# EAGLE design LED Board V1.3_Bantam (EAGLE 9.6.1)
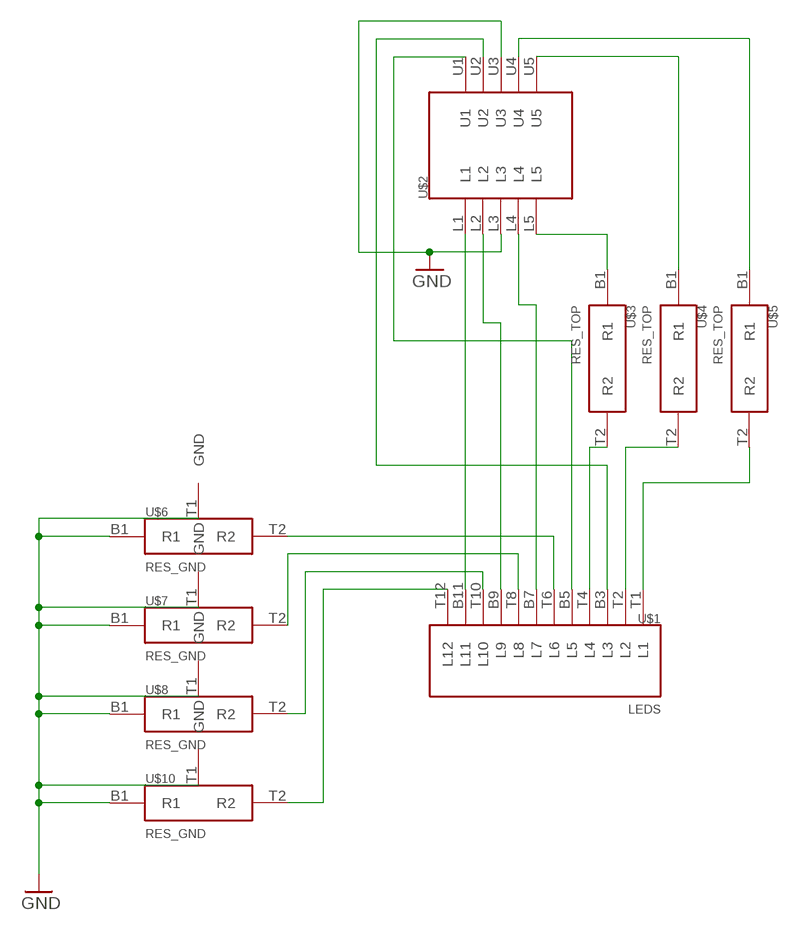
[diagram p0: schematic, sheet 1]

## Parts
U$1  LEDS  [F_LEDS]
U$2  2X5  [F_2X5]
U$3  RES_TOP  [F_RES]
U$4  RES_TOP  [F_RES]
U$5  RES_TOP  [F_RES]
U$6  RES_GND  [F_RES_GND]
U$7  RES_GND  [F_RES_GND]
U$8  RES_GND  [F_RES_GND]
U$10  RES_GND  [F_RES_GND]

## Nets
GND: U$2.L3 U$2.U3 U$6.B1(R1) U$6.T1(GND) U$7.B1(R1) U$7.T1(GND) U$8.B1(R1) U$8.T1(GND) U$10.B1(R1) U$10.T1(GND)
N$1: U$1.T12(L12) U$10.T2(R2)
N$2: U$1.T10(L10) U$8.T2(R2)
N$3: U$1.T8(L8) U$7.T2(R2)
N$4: U$1.T6(L6) U$6.T2(R2)
N$5: U$1.T4(L4) U$3.T2(R2)
N$6: U$1.T2(L2) U$4.T2(R2)
N$7: U$1.T1(L1) U$5.T2(R2)
N$8: U$1.B11(L11) U$2.L1
N$9: U$1.B9(L9) U$2.L2
N$10: U$1.B7(L7) U$2.L4
N$11: U$2.L5 U$3.B1(R1)
N$12: U$2.U5 U$4.B1(R1)
N$13: U$2.U4 U$5.B1(R1)
N$14: U$1.B5(L5) U$2.U1
N$15: U$1.B3(L3) U$2.U2

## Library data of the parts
U$1 = OpenMMS_Bantam:LEDS
U$2 = OpenMMS_Bantam:2X5
U$3-U$5 = OpenMMS_Bantam:RES_TOP
U$6-U$8 U$10 = OpenMMS_Bantam:RES_GND

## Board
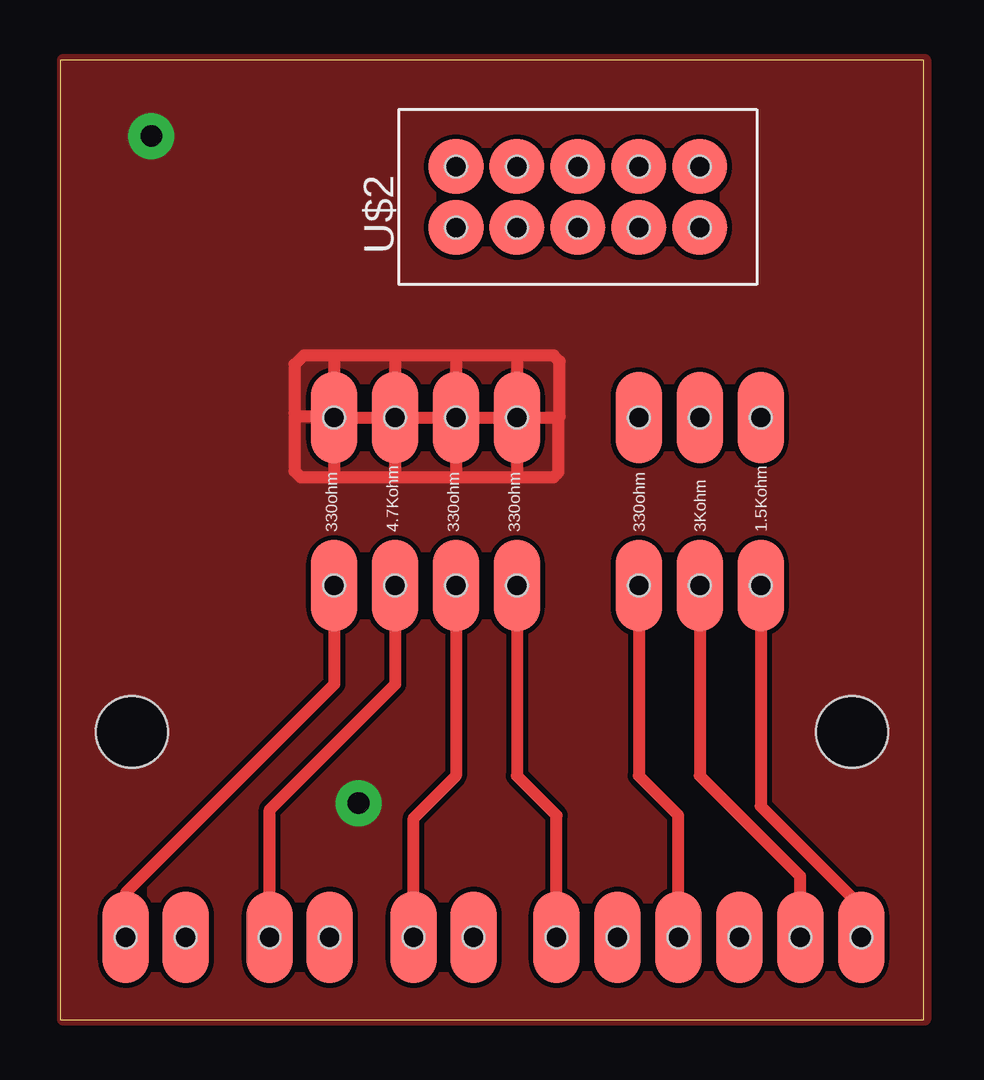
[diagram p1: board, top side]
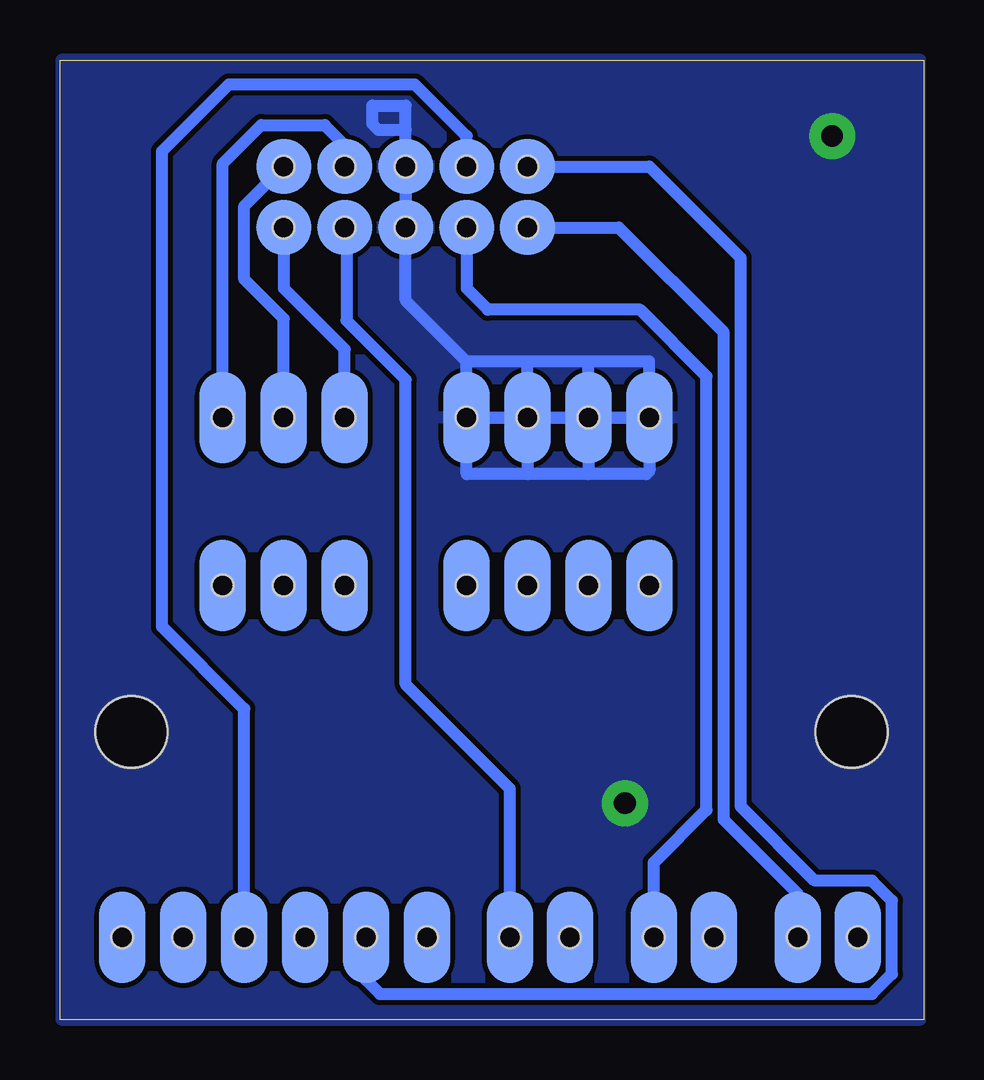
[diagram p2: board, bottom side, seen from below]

Size 36 x 40 mm. Coordinates in mm from the lower left corner, seen from the top.
Outline: 0,0 36,0 36,40 0,40 0,0
Copper layers (1*16): Top 0.035mm / dielectric 1.5mm / Bottom 0.035mm
Design rules "OpenMMS_Bantam": minimum track width 20mil, minimum drill 0.9mm, track to track 8mil, track to pad 8mil, pad to pad 8mil, via to via 8mil, smd to smd 8mil, copper to edge 0mil, drill to drill 0mil, minimum pad ring 20mil, minimum via ring 20mil, stop-mask expansion 4mil, vias tented up to drill 0mil, thermal gap 8mil
Holes 3 mm at 33.02,11.99 3,11.99

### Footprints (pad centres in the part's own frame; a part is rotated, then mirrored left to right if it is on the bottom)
F_LEDS = smd 1.93 x 3.81 bottom: B1 10.16,0; B2 7.62,0; B3 5.08,0; B4 2.54,0; B5 0,0; B6 -2.54,0; B7 -6,0; B8 -8.5,0; B9 -12,0; B10 -14.5,0; B11 -18,0; B12 -20.5,0 | smd 1.93 x 3.81: T1 10.16,0; T2 7.62,0; T3 5.08,0; T4 2.54,0; T5 0,0; T6 -2.54,0; T7 -6,0; T8 -8.5,0; T9 -12,0; T10 -14.5,0; T11 -18,0; T12 -20.5,0 | hole 0.9: 10.16,0; 7.62,0; 5.08,0; 2.54,0; 0,0; -2.54,0; -6,0; -8.5,0; -12,0; -14.5,0; -18,0; -20.5,0
F_2X5 = smd 2.286 x 2.286: B1 -5.08,-1.27; B2 -2.54,-1.27; B3 0,-1.27; B4 2.54,-1.27; B5 5.08,-1.27; B6 5.08,1.27; B7 2.54,1.27; B8 0,1.27; B9 -2.54,1.27; B20 -5.08,1.27 | smd 2.286 x 2.286 bottom: L1 -5.08,-1.27; L2 -2.54,-1.27; L3 0,-1.27; L4 2.54,-1.27; L5 5.08,-1.27; U1 -5.08,1.27; U2 -2.54,1.27; U3 0,1.27; U4 2.54,1.27; U5 5.08,1.27 | hole 0.9: -5.08,-1.27; -2.54,-1.27; 0,-1.27; 2.54,-1.27; 5.08,-1.27; 5.08,1.27; 2.54,1.27; 0,1.27; -2.54,1.27; -5.08,1.27
F_RES = smd 1.93 x 3.81 bottom: B1 0,3.5; B2 0,-3.5 | smd 1.93 x 3.81: T1 0,3.5; T2 0,-3.5 | hole 0.9: 0,3.5; 0,-3.5
F_RES_GND = smd 1.93 x 3.81 bottom: B1 0,3.5; B2 0,-3.5 | smd 1.93 x 3.81: T1 0,3.5; T2 0,-3.5 | hole 0.9: 0,3.5; 0,-3.5

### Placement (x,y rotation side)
U$1  23.24,3.43 0 top
U$2  21.59,34.29 0 top
U$3  24.13,21.59 0 top
U$4  26.67,21.59 0 top
U$5  29.21,21.59 0 top
U$6  19.05,21.59 0 top
U$7  16.51,21.59 0 top
U$8  13.97,21.59 0 top
U$10  11.43,21.59 0 top

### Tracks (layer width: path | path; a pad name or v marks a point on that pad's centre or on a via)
GND  (via drill 0.9)
  Top 0.508: 13.27,25.09 U$10.T1 11.43,22.61 | 13.27,25.09 U$8.T1 | U$8.T1 15.81,25.09 | 15.81,25.09 U$7.T1 | U$7.T1 18.35,25.09 | 18.35,25.09 U$6.T1 | U$6.T1 20.77,25.09 | 20.77,25.09 20.83,25.15 20.83,27.43 20.57,27.69 19.05,27.69 | 19.05,27.69 16.51,27.69 | 16.51,27.69 13.97,27.69 | 13.97,27.69 11.43,27.69 | 11.43,27.69 10.16,27.69 9.78,27.3 9.78,25.27 | 9.78,25.27 9.91,25.15 10.67,25.15 10.73,25.09 10.73,25.38 11.43,26.09 11.43,27.69 | 9.78,25.27 9.78,22.86 10.03,22.61 11.43,22.61 | 11.43,22.61 13.97,22.61 | 13.97,22.61 16.51,22.61 | 16.51,22.61 19.05,22.61 | 19.05,22.61 20.57,22.61 20.77,22.8 20.77,25.09 | 13.27,25.09 13.27,25.38 13.97,26.09 13.97,27.69 | U$8.T1 13.97,22.61 | 15.81,25.09 15.81,25.38 16.51,26.09 16.51,27.69 | U$7.T1 16.51,22.61 | 18.35,25.09 18.35,25.38 19.05,26.09 19.05,27.69 | U$6.T1 19.05,22.61
  Bottom 0.508: 19.05,27.43 U$6.T1 U$7.T1 | 19.05,27.43 21.59,29.97 21.59,32.02 20.89,32.73 20.89,33.02 | U$10.T1 11.43,27.43 13.97,27.43 | 13.97,27.43 16.51,27.43 | 16.51,27.43 19.05,27.43 | U$8.T1 13.97,27.43 | U$7.T1 16.51,27.43 | U$2.L3 U$2.U3 21.59,37.08 | U$10.T1 11.43,22.86 11.56,22.73 13.97,22.73 | 13.97,22.73 16.51,22.73 | 16.51,22.73 19.05,22.73 19.05,24.09 18.35,24.8 18.35,25.09 | U$8.T1 13.97,22.73 | U$7.T1 16.51,22.73 | U$7.T1 U$8.T1 | U$8.T1 U$10.T1 | 21.59,37.08 21.59,38.1 22.99,38.1 22.99,37.34 22.73,37.08 21.59,37.08
  other vias: 3.81,36.83 12.45,9.02
  pour Top: 0.13,40.01 36.07,40.01 36.07,0 0.13,0
  pour Bottom: 0.13,40.01 35.94,40.01 35.94,0 0.13,0
N$1
  Top 0.508: U$1.T12 2.74,5.28 11.43,13.97 U$10.T2
N$2
  Top 0.508: U$1.T10 8.74,8.74 13.97,13.97 U$8.T2
N$3
  Top 0.508: U$1.T8 14.74,8.39 16.51,10.16 U$7.T2
N$4
  Top 0.508: U$1.T6 20.7,8.51 19.05,10.16 U$6.T2
N$5
  Top 0.508: U$1.T4 25.78,8.51 24.13,10.16 U$3.T2
N$6
  Top 0.508: U$1.T2 30.86,5.97 26.67,10.16 U$4.T2
N$7
  Top 0.508: U$1.T1 33.4,4.7 29.21,8.89 U$5.T2
N$8
  Bottom 0.508: U$1.B11 5.24,5.24 8.33,8.33 8.33,28.65 12.7,33.02 U$2.L1
N$9
  Bottom 0.508: U$1.B9 11.24,6.54 9.04,8.74 9.04,26.82 11.81,29.59 18.16,29.59 19.05,30.48 U$2.L2
N$10
  Bottom 0.508: U$1.B7 17.24,9.62 21.59,13.97 21.59,26.67 24.06,29.14 24.06,33.02 U$2.L4
N$11
  Bottom 0.508: U$3.B1 24.13,27.94 26.67,30.48 U$2.L5
N$12
  Bottom 0.508: U$4.B1 26.67,29.21 28.32,30.86 28.32,33.91 U$2.U5
N$13
  Bottom 0.508: U$5.B1 29.21,35.69 27.61,37.29 24.97,37.29 24.13,36.45 U$2.U4
N$14
  Bottom 0.508: U$1.B5 23.24,1.65 22.66,1.07 2.15,1.07 1.32,1.9 1.32,4.96 2.15,5.79 4.52,5.79 7.62,8.89 7.62,31.75 11.43,35.56 U$2.U1
N$15
  Bottom 0.508: U$1.B3 28.32,12.95 31.75,16.38 31.75,36.2 28.96,38.99 21.21,38.99 19.05,36.83 U$2.U2

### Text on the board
tPlace: 330ohm | 4.7Kohm | 330ohm | 330ohm | 330ohm | 3Kohm | 1.5Kohm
